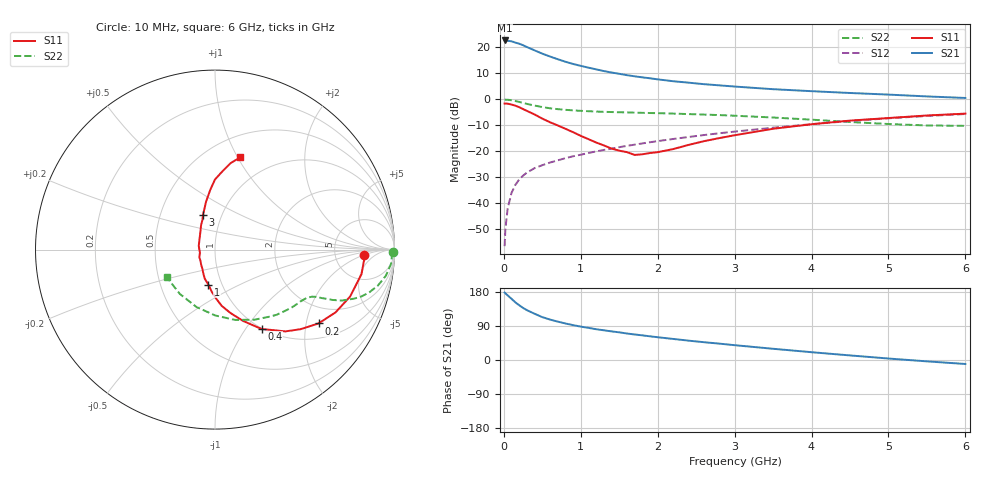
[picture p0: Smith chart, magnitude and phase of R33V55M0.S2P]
! SIEMENS Small Signal Semiconductors
! BFR181
! Si NPN RF Bipolar Junction Transistor in SOT23
! VCE = 3.5 V  IC = 5 mA
! Common Emitter S-Parameters:  May  1996
# GHz  S  MA  R  50
!  f  S11  S21  S12  S22
! GHz  MAG  ANG  MAG  ANG  MAG  ANG  MAG  ANG
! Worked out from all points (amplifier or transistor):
!   36 points, 10 MHz to 6 GHz, reference 50 ohm
!   highest |S21| = 22.7 dB at 10 MHz (marker M1)
!   |S21| within 3 dB of that: start of sweep to 335.9 MHz
!   unconditionally stable (mu >= 1): 1.137 GHz to 2.959 GHz
!   at 250 MHz: K = 0.41, MSG = 25.1 dB, |S12| = -29.3 dB
!   at 1.4 GHz: K = 1.05, MAG = 13.3 dB, |S12| = -18.9 dB
!   at 6 GHz: K = 0.86, MSG = 3.1 dB, |S12| = -5.6 dB
!   lowest NFmin = 1.55 dB at 450 MHz
!   S11 on the Smith chart (normalised r, x): 10 MHz: 10, -2; 200 MHz: 1.43, -2.36; 400 MHz: 0.99, -1.19; 1 GHz: 0.86, -0.35; 3 GHz: 0.82, +0.33; 6 GHz: 0.71, +1.02
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0.01  0.8323 -2.2  13.62 177.9  0.0015 87.3  0.9924 -0.9
0.02  0.8331 -3.7  13.43 175.9  0.0032 89.0  0.9866 -1.8
0.05  0.8277 -9.5  13.43 170.5  0.008 84.9  0.9846 -4.5
0.1  0.7967 -19.2  13.11 161.4  0.0159 79.3  0.9637 -8.6
0.15  0.7573 -27.5  12.38 152.1  0.0227 75.7  0.9302 -12.4
0.2  0.7084 -35.5  11.78 144.5  0.0289 72.3  0.8942 -15.3
0.25  0.6514 -42.9  11.02 137.4  0.0341 69.6  0.8561 -17.8
0.3  0.6011 -49.3  10.17 131.5  0.0391 67.9  0.8196 -19.5
0.4  0.5127 -59.6  8.771 122.0  0.0476 64.8  0.761 -21.9
0.5  0.4271 -68.5  7.587 113.1  0.0542 63.6  0.712 -23.2
0.6  0.3636 -76.3  6.689 106.7  0.0609 63.1  0.6752 -23.9
0.8  0.2722 -88.8  5.306 96.4  0.0739 63.1  0.6302 -24.9
1  0.1989 -100.6  4.416 88.1  0.0863 63.7  0.6024 -25.8
1.1  0.172 -109.3  4.084 84.8  0.0931 64.2  0.5928 -26.5
1.3  0.1303 -122.3  3.51 78.4  0.1065 64.4  0.5765 -27.8
1.6  0.0967 -154.9  2.924 69.9  0.1276 64.3  0.5609 -30.5
2.2  0.1105 140.1  2.239 55.6  0.1731 62.7  0.533 -37.7
3  0.2044 109.1  1.767 39.1  0.2401 58.1  0.4851 -50.1
3.5  0.2722 100.5  1.572 29.6  0.2854 54.1  0.4483 -60.6
4.5  0.391 90.0  1.329 12.1  0.3837 43.9  0.3671 -89.8
5.5  0.4904 79.7  1.141 -3.6  0.4795 31.3  0.3152 -128.5
6  0.5324 74.7  1.066 -10.5  0.5235 24.3  0.3097 -149.9
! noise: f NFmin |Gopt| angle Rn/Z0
0.45  1.55  0.48  17  0.36
0.9  1.65  0.4  35  0.34
1.8  2  0.18  88  0.34
